(* Logix 5000 AddOnInstructionDefinition export Banner_RSio_ISD_Baseline_Info_v1; software revision 33.00 *)

TYPE Banner_RSio_ISD_Baseline_v1 :
STRUCT
   AccessChain : SINT;
   BaselineInfo : SINT[40];
END_STRUCT
END_TYPE

ADD_ON_INSTRUCTION Banner_RSio_ISD_Baseline_Info_v1   (* revision 1.0 *)
VAR_IN_OUT
   Baseline : Banner_RSio_ISD_Baseline_v1; {required}
   MSG : MESSAGE; {required}
   Activate : BOOL; {required}
END_VAR
VAR_OUTPUT
   Busy : BOOL; {visible}
   Done : BOOL; {visible}
   Error : BOOL; {visible}
END_VAR
VAR
   Timer : TIMER := (PRE := 5000); {access None}
   Control : DINT; {access None}
END_VAR

ROUTINE Logic   (* ladder *)
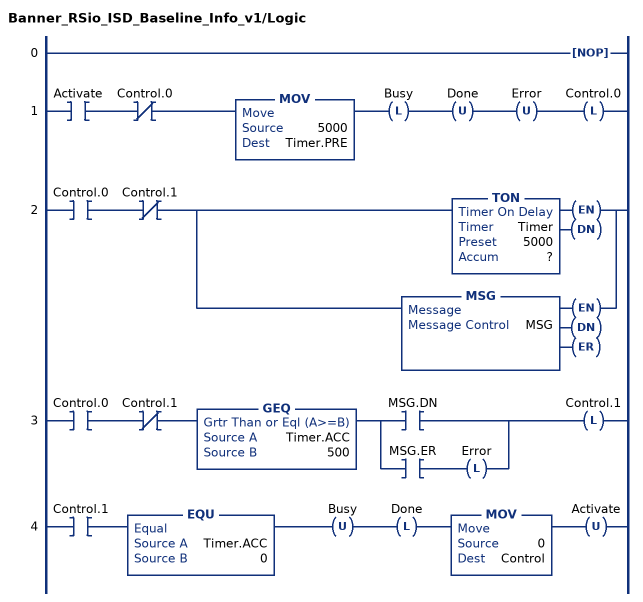
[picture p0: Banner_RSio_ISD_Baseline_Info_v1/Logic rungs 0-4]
   0: NOP();
   1: XIC(Activate)XIO(Control.0)MOV(5000,Timer.PRE)OTL(Busy)OTU(Done)OTU(Error)OTL(Control.0);
   2: XIC(Control.0)XIO(Control.1)[TON(Timer,?,?) ,MSG(MSG) ];
   3: XIC(Control.0)XIO(Control.1)GEQ(Timer.ACC,500)[XIC(MSG.DN) ,XIC(MSG.ER) OTL(Error) ]OTL(Control.1);
   4: XIC(Control.1)EQU(Timer.ACC,0)OTU(Busy)OTL(Done)MOV(0,Control)OTU(Activate);
END_ROUTINE
END_ADD_ON_INSTRUCTION
